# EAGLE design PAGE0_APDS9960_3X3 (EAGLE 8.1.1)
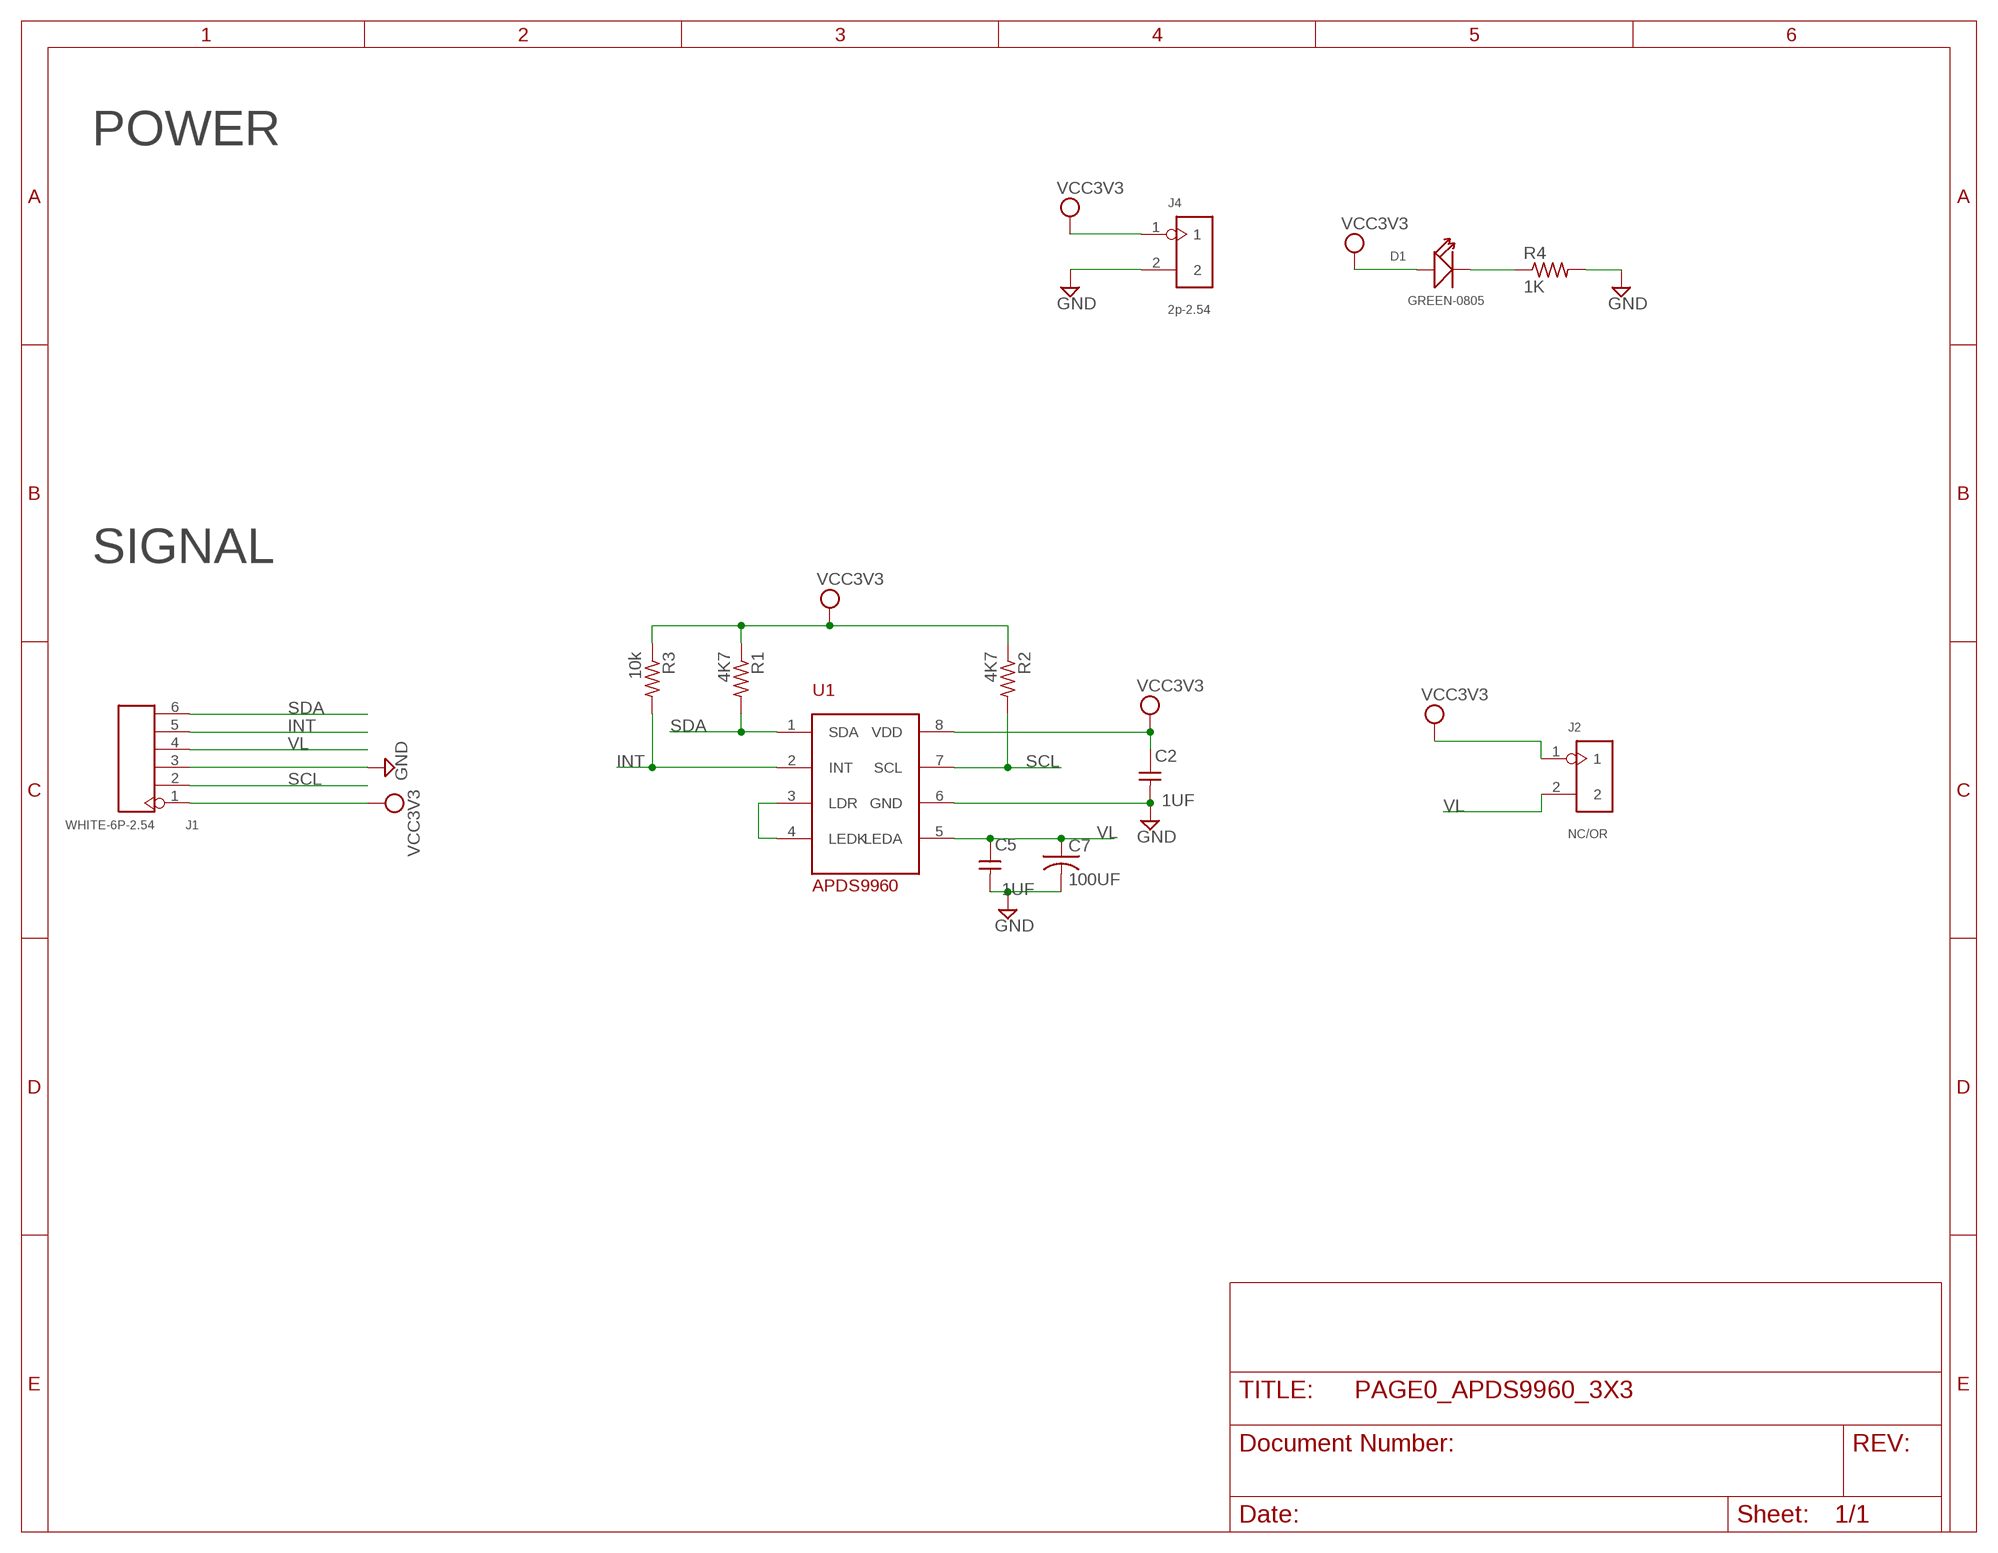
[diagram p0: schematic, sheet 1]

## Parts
C2  1UF  CAP-UNPOLARIZEDFAB  [C1206FAB]
C5  1UF  CAP-UNPOLARIZEDFAB  [C1206FAB]
C7  100UF  C-USC1210  [C1210]
D1  GREEN-0805  SMD-LED-CLEAR-GREEN(0805)  [LED-0805]
J1  WHITE-6P-2.54  DIP-WHITE-MALE-HEADER-VERT(6P-2.54)  [H6-2.54]
J2  NC/OR  DIP-BLUE-MALE-HEADER-VERT(2P-2.54)  [H2-2.54]
J4  2p-2.54  DIP-BLUE-MALE-HEADER-VERT(2P-2.54)  [H2-2.54]
R1  4K7  RES-US1206FAB  [R1206FAB]
R2  4K7  RES-US1206FAB  [R1206FAB]
R3  10k  RES-US1206FAB  [R1206FAB]
R4  1K  RES-US1206FAB  [R1206FAB]
U1  APDS9960  [APDS9960_8PIN_NEW]

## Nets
GND: C2.2 C5.2 C7.2 J1.3 J4.2 R4.2 U1.6(GND)
INT: J1.5 R3.2 U1.2(INT)
N$1: D1.- R4.1
N$3: U1.3(LDR) U1.4(LEDK)
SCL: J1.2 R2.2 U1.7(SCL)
SDA: J1.6 R1.2 U1.1(SDA)
VCC: C2.1 D1.+ J1.1 J2.1 J4.1 R1.1 R2.1 R3.1 U1.8(VDD) ; supply symbol labelled VCC3V3
VL: C5.1 C7.1 J1.4 J2.2 U1.5(LEDA)

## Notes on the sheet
- POWER
- SIGNAL

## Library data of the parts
C2 C5 = fab:CAP-UNPOLARIZED
C7 = rcl:C-US: CAPACITOR, American symbol
D1 = Seeed-OPL-Diode:SMD-LED-CLEAR-GREEN(0805): 304090057; MPN: 17-215SYGC/S530-E2/TR8
J1 = Seeed-OPL-Connector:DIP-WHITE-MALE-HEADER-VERT(6P-2.54): 320020022; MPN: P125-1106A0BS116A2
J2 = Seeed-OPL-Connector:DIP-BLUE-MALE-HEADER-VERT(2P-2.54): 320020015; MPN: P125-1102A0BS116A2; VALUE: 2p-2.54
J4 = Seeed-OPL-Connector:DIP-BLUE-MALE-HEADER-VERT(2P-2.54): 320020015; MPN: P125-1102A0BS116A2
R1-R4 = fab:RES-US: Resistor (US Symbol)
U1 = APDS9960:APDS9960: APDS9960 手势传感器

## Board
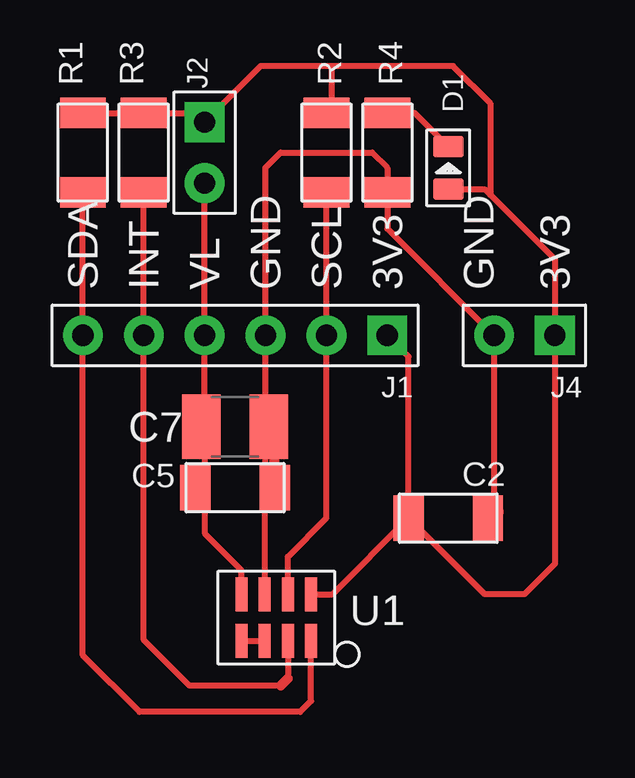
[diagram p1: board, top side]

No outline drawn. Coordinates in mm, seen from the top.
Copper layers (1*16): Top 0.035mm / dielectric 1.5mm / Bottom 0.035mm
Design rules "default": minimum track width 10mil, minimum drill 24mil, track to track 8mil, track to pad 8mil, pad to pad 8mil, via to via 8mil, smd to smd 8mil, copper to edge 40mil, drill to drill 8mil, minimum pad ring 10mil, minimum via ring 8mil, stop-mask expansion 4mil, vias tented up to drill 0mil, thermal gap 10mil

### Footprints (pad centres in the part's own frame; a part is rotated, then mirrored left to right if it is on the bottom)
C1206FAB = smd 1.27 x 1.905: 1 -1.651,0; 2 1.651,0
C1210 = smd 1.6 x 2.7: 1 -1.4,0; 2 1.4,0
LED-0805 = smd 0.889 x 1.27: + -0.889,0; - 0.889,0
H6-2.54 = drill 0.889 pad 1.651 square: 1 0,6.35 | drill 0.889 pad 1.651: 2 0,3.81; 3 0,1.27; 4 0,-1.27; 5 0,-3.81; 6 0,-6.35
H2-2.54 = drill 0.889 pad 1.651 square: 1 0,1.27 | drill 0.889 pad 1.651: 2 0,-1.27
R1206FAB = smd 1.27 x 1.905: 1 -1.651,0; 2 1.651,0
APDS9960_8PIN_NEW = smd 1.422 x 0.5: 1 1.94,0; 2 1.94,-0.97; 3 1.94,-1.94; 4 1.94,-2.91; 5 0,-2.91; 6 0,-1.94; 7 0,-0.97; 8 0,0

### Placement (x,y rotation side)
C2  22.23,9.53 0 top
C5  13.34,10.79 0 top
C7  13.34,13.34 0 top
D1  22.23,24.13 90 top
J1  13.34,17.14 270 top
J2  12.06,24.77 0 top
J4  25.4,17.14 270 top
R1  6.99,24.77 270 top
R2  17.14,24.77 270 top
R3  9.53,24.77 270 top
R4  19.68,24.77 270 top
U1  16.51,6.35 270 top

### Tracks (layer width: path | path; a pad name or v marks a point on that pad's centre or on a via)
GND
  Top 0.254: 14.57,10.16 U1.6 | 14.61,10.2 J1.3 14.61,24.13 15.24,24.77 19.05,24.77 19.68,24.13 R4.2 19.68,21.59 J4.2 24.13,9.78
  Top 0.406: C7.2 14.99,13.08 C5.2 14.57,10.38 14.57,10.16 14.61,10.2
  Top 0.813: 24.13,9.78 C2.2
INT
  Top 0.254: U1.2 15.54,2.84 | 15.24,2.54 11.43,2.54 9.53,4.45 J1.5 R3.2
  Top 0.406: 15.54,2.84 15.24,2.54
N$1
  Top 0.254: R4.1 20.83,26.42 D1.-
N$3
  Top 0.254: U1.4 U1.3
SCL
  Top 0.254: U1.7 15.54,7.92 17.14,9.53 J1.2 R2.2
SDA
  Top 0.254: U1.1 16.51,1.91 16.05,1.45 9.35,1.45 6.99,3.81 J1.6 R1.2
VCC
  Top 0.254: 17.35,28.37 22.43,28.37 23.98,26.82 23.98,23.01 | 17.35,28.37 17.35,26.62 | 17.35,28.37 14.4,28.37 J2.1 | R1.1 R3.1 11.68,26.42 | 23.98,23.01 26.67,20.32 J4.1 26.67,7.62 25.4,6.35 23.75,6.35 C2.1 | D1.+ 23.75,23.24 23.98,23.01 | C2.1 20.57,16.26 J1.1 | U1.8 17.4,6.35 C2.1
  Top 0.813: 17.35,26.62 R2.1 | 11.68,26.42 J2.1
VL
  Top 0.254: U1.5 13.6,7.36 12.06,8.89 12.06,10.79 12.06,13.34 J1.4 J2.2
  Top 0.406: C5.1 12.06,10.79 | C7.1 12.06,13.34

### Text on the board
tNames: SDA | INT | VL | GND | SCL | 3V3 | GND | 3V3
